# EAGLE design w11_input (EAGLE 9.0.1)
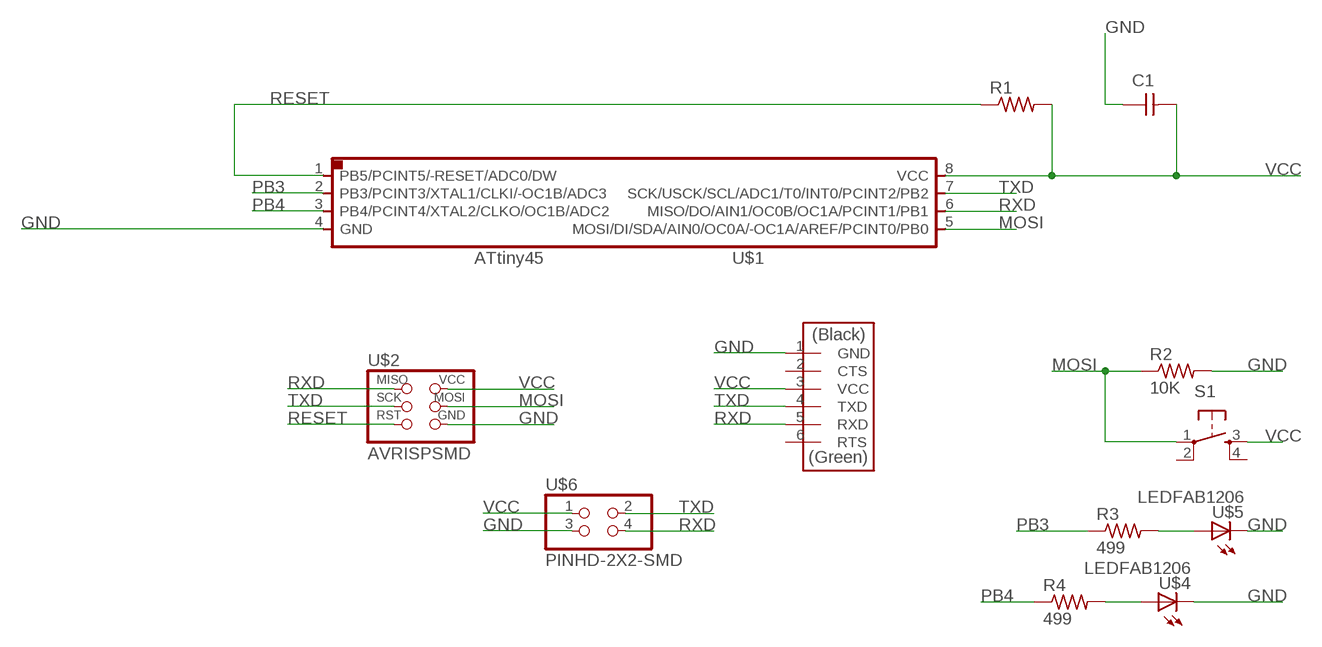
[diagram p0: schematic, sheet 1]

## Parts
C1  CAP-UNPOLARIZEDFAB  [C1206FAB]
R1  RES-US1206FAB  [R1206FAB]
R2  10K  RES-US1206FAB  [R1206FAB]
R3  499  RES-US1206FAB  [R1206FAB]
R4  499  RES-US1206FAB  [R1206FAB]
S1  6MM_SWITCH6MM_SWITCH  [6MM_SWITCH]
U$1  ATTINY45SI  [SOIC8]
U$2  AVRISPSMD  [2X03SMD]
U$3  FTDI-SMD-HEADER  [1X06SMD]
U$4  LEDFAB1206  [LED1206FAB]
U$5  LEDFAB1206  [LED1206FAB]
U$6  PINHD-2X2-SMD  [2X02SMD]

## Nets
GND: C1.1 R2.2 U$1.4(GND) U$2.6(GND) U$3.1(GND) U$4.2(C) U$5.2(C) U$6.3
MOSI: R2.1 S1.1(P) U$1.5(MOSI/DI/SDA/AIN0/OC0A/-OC1A/AREF/PCINT0/PB0) U$2.4(MOSI)
N$15: R4.2 U$4.1(A)
N$16: R3.2 U$5.1(A)
PB3: R3.1 U$1.2(PB3/PCINT3/XTAL1/CLKI/-OC1B/ADC3)
PB4: R4.1 U$1.3(PB4/PCINT4/XTAL2/CLKO/OC1B/ADC2)
RESET: R1.1 U$1.1(PB5/PCINT5/-RESET/ADC0/DW) U$2.5(RST)
RXD: U$1.6(MISO/DO/AIN1/OC0B/OC1A/PCINT1/PB1) U$2.1(MISO) U$3.5(RXD) U$6.4
TXD: U$1.7(SCK/USCK/SCL/ADC1/T0/INT0/PCINT2/PB2) U$2.3(SCK) U$3.4(TXD) U$6.2
VCC: C1.2 R1.2 S1.3(S) U$1.8(VCC) U$2.2(VCC) U$3.3(VCC) U$6.1
Unconnected: S1.2(P1) S1.4(S1) U$3.2(CTS) U$3.6(RTS)

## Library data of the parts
C1 = fab:CAP-UNPOLARIZED
R1-R4 = fab:RES-US: Resistor (US Symbol)
S1 = fab:6MM_SWITCH: OMRON SWITCH
U$1 = fab:ATTINY45
U$2 = fab:AVRISP
U$3 = fab:FTDI-SMD-HEADER
U$4 U$5 = fab:LED: LED
U$6 = fab:PINHD-2X2-SMD

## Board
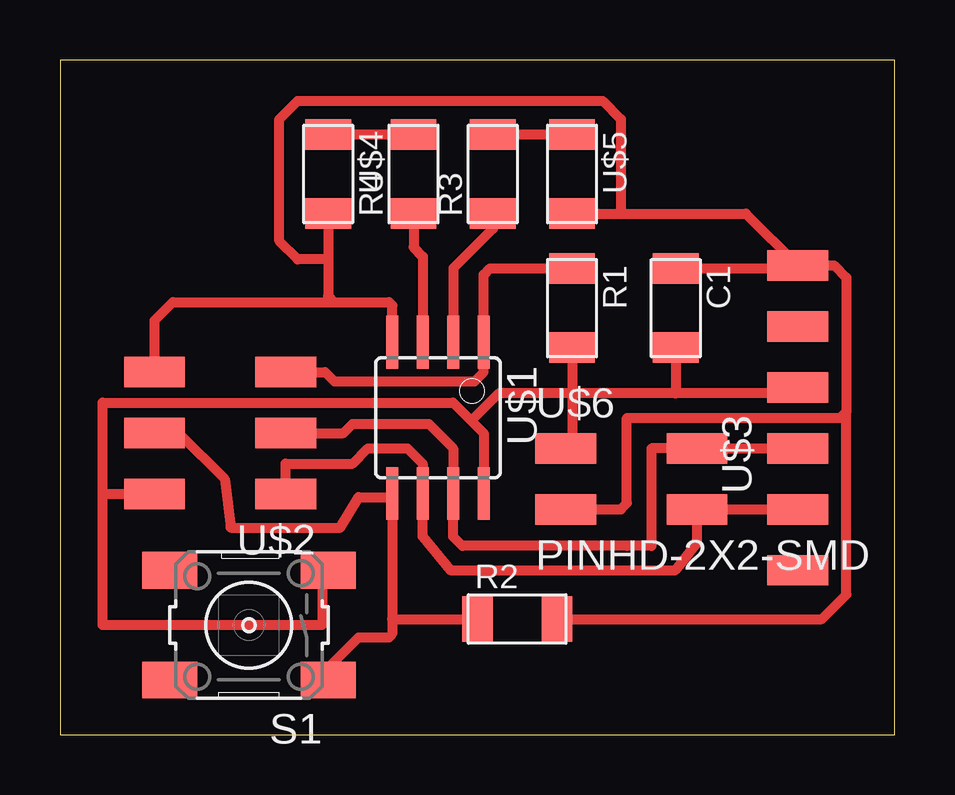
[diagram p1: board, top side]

Size 34.78 x 28.12 mm. Coordinates in mm from the lower left corner, seen from the top.
Outline: 0,0 34.78,0 34.78,28.12 0,28.12 0,0
Copper layers (1*16): Top 0.035mm / dielectric 1.5mm / Bottom 0.035mm
Design rules "default": minimum track width 6mil, minimum drill 0.35mm, track to track 6mil, track to pad 6mil, pad to pad 6mil, via to via 6mil, smd to smd 6mil, copper to edge 40mil, drill to drill 6mil, minimum pad ring 10mil, minimum via ring 8mil, stop-mask expansion 4mil, vias tented up to drill 0mil, thermal gap 10mil

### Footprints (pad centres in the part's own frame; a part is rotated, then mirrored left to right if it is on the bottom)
C1206FAB = smd 1.27 x 1.905: 1 -1.651,0; 2 1.651,0
R1206FAB = smd 1.27 x 1.905: 1 -1.651,0; 2 1.651,0
6MM_SWITCH = smd 2.286 x 1.524: 1 -3.302,2.286; 2 3.302,2.286; 3 -3.302,-2.286; 4 3.302,-2.286
SOIC8 = smd 0.5 x 2.2: 1 -1.905,-3.154; 2 -0.645,-3.154; 3 0.625,-3.154; 4 1.895,-3.154; 5 1.905,3.154; 6 0.635,3.154; 7 -0.635,3.154; 8 -1.905,3.154
2X03SMD = smd 2.54 x 1.27: 1 -2.54,2.54; 2 2.92,2.54; 3 -2.54,0; 4 2.92,0; 5 -2.54,-2.54; 6 2.92,-2.54
1X06SMD = smd 2.54 x 1.27: 1 0,6.35; 2 0,3.81; 3 0,1.27; 4 0,-1.27; 5 0,-3.81; 6 0,-6.35
LED1206FAB = smd 1.27 x 1.905: 1 -1.651,0; 2 1.651,0
2X02SMD = smd 2.54 x 1.27: 1 -2.54,1.27; 2 2.92,1.27; 3 -2.54,-1.27; 4 2.92,-1.27

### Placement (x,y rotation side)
C1  25.65,17.78 270 top
R1  21.34,17.78 270 top
R2  19.05,4.83 0 top
R3  18.03,23.37 90 top
R4  14.73,23.37 90 top
S1  7.87,4.57 180 top
U$1  15.75,13.21 180 top
U$2  6.86,12.57 180 top
U$3  30.73,13.21 0 top
U$4  11.18,23.37 270 top
U$5  21.34,23.37 270 top
U$6  23.62,10.67 0 top

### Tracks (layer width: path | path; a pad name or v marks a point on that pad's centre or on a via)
GND
  Top 0.406: U$1.4 13.85,17.9 13.72,18.03 11.43,18.03 | U$2.6 3.94,17.27 4.7,18.03 11.43,18.03 | U$6.3 23.37,9.4 23.62,9.65 23.62,13.21 32.51,13.21 32.77,13.46 | 32.77,13.46 32.77,19.05 32.26,19.56 U$3.1 | 32.77,13.46 32.77,5.84 31.75,4.83 R2.2 | U$4.2 11.18,19.81 | 11.18,19.81 11.18,18.29 11.43,18.03 | 21.46,21.59 U$5.2 23.37,21.72 | 23.37,21.72 28.57,21.72 U$3.1 | C1.1 30.61,19.43 U$3.1 | 11.18,19.81 9.91,19.81 9.14,20.57 9.14,25.65 9.91,26.42 22.61,26.42 23.37,25.65 23.37,21.72
MOSI
  Top 0.406: U$2.4 4.95,12.57 6.86,10.67 7.11,8.64 11.68,8.64 12.45,9.91 13.84,9.91 | U$1.5 13.84,9.91 | 13.84,9.91 13.84,4.83 | 13.84,4.83 13.84,4.19 13.72,4.06 12.45,4.06 11.18,2.79 S1.1 | 13.84,4.83 R2.1
N$15
  Top 0.406: U$4.1 R4.2
N$16
  Top 0.406: R3.2 U$5.1
PB3
  Top 0.406: R3.1 18.03,21.08 16.39,19.44 U$1.2
PB4
  Top 0.406: R4.1 14.73,20.32 15.12,19.93 U$1.3
RESET
  Top 0.406: U$2.5 11.05,15.11 11.43,14.73 17.27,14.73 17.65,15.11 U$1.1 17.65,19.18 17.91,19.43 R1.1
RXD
  Top 0.406: U$3.5 U$6.4 26.54,8 25.65,6.86 16.26,6.86 15.11,8.25 U$1.6 15.11,11.3 14.48,11.94 12.83,11.94 12.19,11.3 9.4,11.3 U$2.1
TXD
  Top 0.406: U$3.4 U$6.2 24.64,11.94 24.64,7.87 23.62,7.87 16.76,7.87 16.38,8.25 U$1.7 16.38,11.94 15.37,12.95 12.19,12.95 11.81,12.57 U$2.3
VCC
  Top 0.406: U$2.2 1.78,10.03 | 1.78,10.03 1.78,13.84 16.38,13.84 17.15,13.08 | 17.15,13.08 17.65,12.57 U$1.8 | U$3.3 30.48,14.22 25.65,14.22 | 17.15,13.08 18.29,14.22 21.34,14.22 | 25.65,14.22 21.34,14.22 | R1.2 21.34,14.22 | 21.34,14.22 21.34,12.19 U$6.1 | S1.3 10.92,6.6 10.92,4.57 1.78,4.57 1.78,10.03 | C1.2 25.65,14.22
